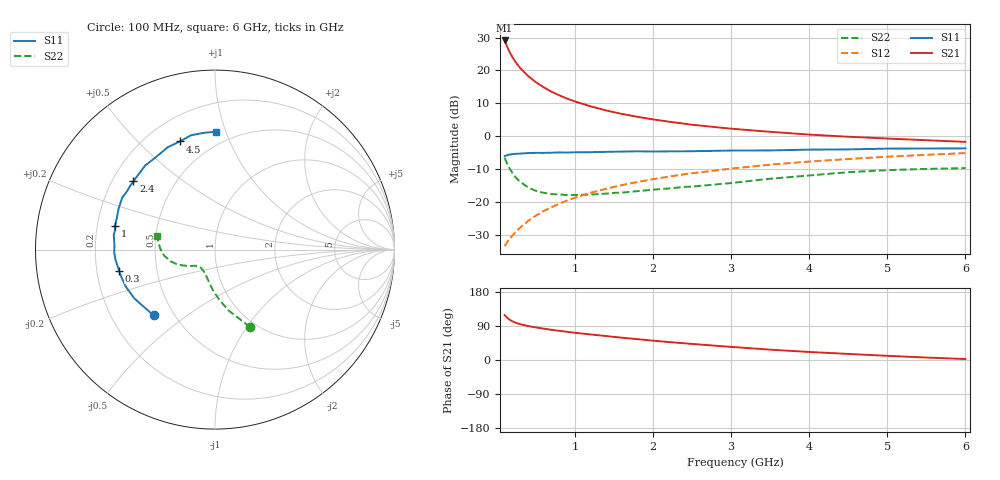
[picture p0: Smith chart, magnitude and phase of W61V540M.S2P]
! SIEMENS Small Signal Semiconductors
! BFR193W
! Si NPN RF Bipolar Junction Transistor in SOT323
! VCE = 1.5 V  IC = 40 mA
! Common Emitter S-Parameters:  September  1992
# GHz  S  MA  R  50
!  f  S11  S21  S12  S22
! GHz  MAG  ANG  MAG  ANG  MAG  ANG  MAG  ANG
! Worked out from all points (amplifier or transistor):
!   28 points, 100 MHz to 6 GHz, reference 50 ohm
!   highest |S21| = 29.1 dB at 100 MHz (marker M1)
!   |S21| within 3 dB of that: start of sweep to 153.2 MHz
!   unconditionally stable (mu >= 1): 473.9 MHz to 2.607 GHz
!   at 300 MHz: K = 0.92, MSG = 24.2 dB, |S12| = -27.7 dB
!   at 1.5 GHz: K = 1.04, MAG = 10.1 dB, |S12| = -15.4 dB
!   at 6 GHz: K = 0.94, MSG = 1.7 dB, |S12| = -5.1 dB
!   S11 on the Smith chart (normalised r, x): 100 MHz: 0.39, -0.38; 300 MHz: 0.30, -0.10; 1 GHz: 0.28, +0.11; 2.4 GHz: 0.29, +0.34; 4.5 GHz: 0.33, +0.67; 6 GHz: 0.40, +0.93
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0.1  0.5014 -133.1  28.56 118.4  0.0215 57.5  0.4728 -65.7
0.15  0.5256 -148.9  20.55 108.3  0.0265 59.0  0.3469 -77.5
0.2  0.5384 -157.6  15.91 102.0  0.0312 61.0  0.2774 -85.5
0.25  0.5431 -163.2  12.92 97.9  0.0363 63.4  0.2319 -92.1
0.3  0.547 -167.6  10.89 94.5  0.0412 65.3  0.204 -96.5
0.4  0.5572 -174.0  8.242 89.7  0.0517 68.0  0.1677 -104.5
0.5  0.5616 -178.4  6.639 86.0  0.0624 69.8  0.1484 -110.6
0.6  0.5605 177.8  5.558 82.7  0.0734 70.5  0.1389 -116.2
0.7  0.5646 174.8  4.763 79.7  0.084 71.1  0.133 -119.8
0.8  0.57 171.8  4.195 76.9  0.0951 71.1  0.1311 -123.3
0.9  0.5673 169.3  3.737 74.4  0.1061 71.1  0.1282 -126.1
1  0.5727 166.9  3.39 71.8  0.117 70.9  0.1287 -128.2
1.2  0.5747 162.1  2.854 67.5  0.1388 70.0  0.1308 -133.4
1.4  0.5815 158.1  2.474 63.2  0.16 68.8  0.135 -136.6
1.6  0.5863 154.3  2.194 58.9  0.1814 67.6  0.1396 -139.7
2.2  0.5911 143.2  1.671 47.5  0.2444 63.0  0.1615 -145.5
2.4  0.5929 140.0  1.557 44.1  0.265 61.3  0.1707 -147.4
3  0.6087 129.8  1.307 34.6  0.3237 55.9  0.1954 -152.9
3.5  0.6111 122.8  1.171 27.3  0.3715 51.3  0.2269 -158.7
4.5  0.6334 107.9  0.986 16.0  0.4523 42.0  0.2856 -173.2
5.5  0.6539 95.0  0.873 6.5  0.5241 33.1  0.3205 171.3
6  0.6566 89.3  0.824 2.6  0.5564 28.5  0.3293 166.7
